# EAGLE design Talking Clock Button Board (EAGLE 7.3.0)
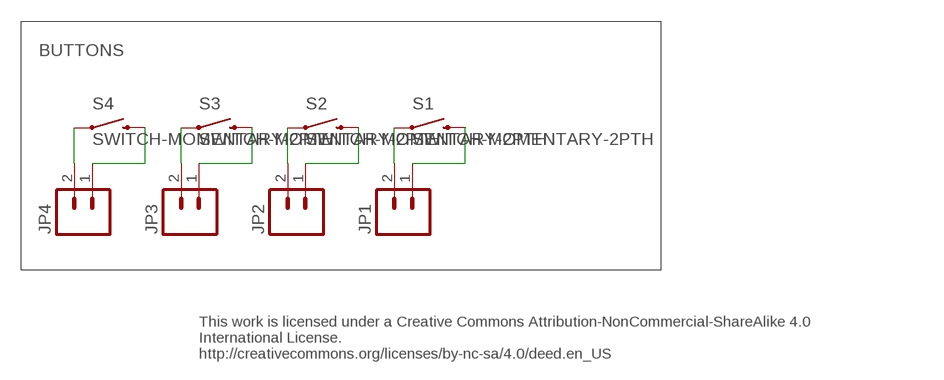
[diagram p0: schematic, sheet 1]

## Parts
JP1  M02PTH  [1X02]
JP2  M02PTH  [1X02]
JP3  M02PTH  [1X02]
JP4  M02PTH  [1X02]
S1  SWITCH-MOMENTARY-2PTH  [TACTILE-PTH]
S2  SWITCH-MOMENTARY-2PTH  [TACTILE-PTH]
S3  SWITCH-MOMENTARY-2PTH  [TACTILE-PTH]
S4  SWITCH-MOMENTARY-2PTH  [TACTILE-PTH]

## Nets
N$1: JP4.2 S4.1
N$2: JP4.1 S4.3
N$3: JP3.2 S3.1
N$4: JP3.1 S3.3
N$5: JP2.2 S2.1
N$6: JP2.1 S2.3
N$7: JP1.2 S1.1
N$8: JP1.1 S1.3

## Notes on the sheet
- BUTTONS
- This work is licensed under a Creative Commons Attribution-NonCommercial-ShareAlike 4.0
  International License.
  http://creativecommons.org/licenses/by-nc-sa/4.0/deed.en_US

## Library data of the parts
JP1-JP4 = SparkFun-Connectors:M02: Standard 2-pin 0.1" header. Use with
S1-S4 = SparkFun-Electromechanical:SWITCH-MOMENTARY-2: Various NO switches- pushbuttons, reed, etc; PROD_ID: SWCH-08441

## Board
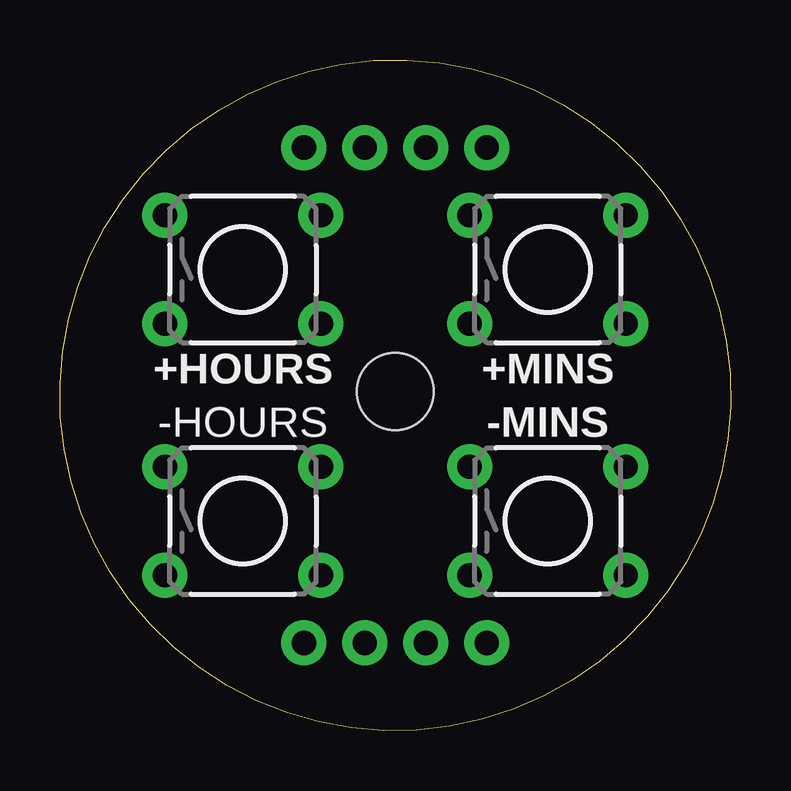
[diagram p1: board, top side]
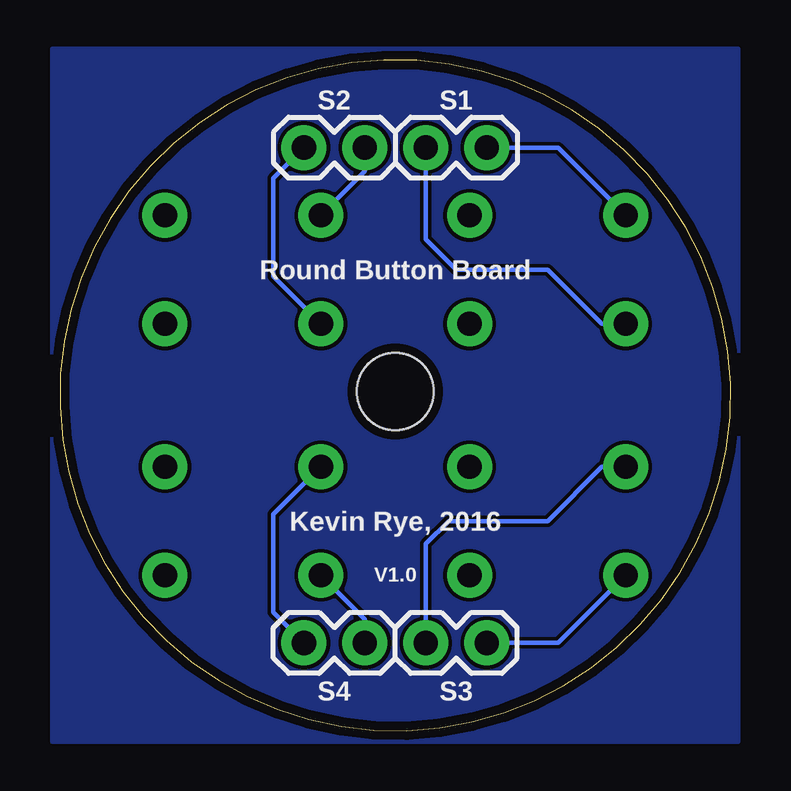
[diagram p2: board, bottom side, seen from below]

Size 27.94 x 27.94 mm. Coordinates in mm from the lower left corner, seen from the top.
Outline: 0,14.45 arc-180 27.94,13.49 arc-180 0,14.45
Copper layers (1*16): Top 0.0356mm / dielectric 1.5011mm / Bottom 0.0356mm
Design rules "oshpark-2layer": minimum track width 6mil, minimum drill 13mil, track to track 6mil, track to pad 6mil, pad to pad 6mil, via to via 6mil, smd to smd 6mil, copper to edge 15mil, drill to drill 6mil, minimum pad ring 7mil, minimum via ring 7mil, stop-mask expansion 2.5mil, vias tented up to drill 0mil, thermal gap 10mil
Holes 3.2 mm at 13.97,14.13

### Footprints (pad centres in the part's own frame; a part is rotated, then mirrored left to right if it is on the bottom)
1X02 = drill 1.016 pad 1.88: 1 0,0; 2 2.54,0
TACTILE-PTH = drill 1.016 pad 1.88: 1 -3.251,2.261; 2 3.251,2.261; 3 -3.251,-2.261; 4 3.251,-2.261

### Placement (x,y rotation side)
JP1  12.7,24.29 0 bottom
JP2  17.78,24.29 0 bottom
JP3  10.16,3.65 180 bottom
JP4  15.24,3.65 180 bottom
S1  7.62,19.21 0 top
S2  20.32,19.21 0 top
S3  7.62,8.73 0 top
S4  20.32,8.73 0 top

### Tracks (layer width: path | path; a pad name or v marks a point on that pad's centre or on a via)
GND
  pour Bottom: -0.32,28.42 28.26,28.42 28.26,-0.48 -0.32,-0.48
N$1
  Bottom 0.178: JP4.2 19.05,4.92 19.05,9.01 S4.1
N$2
  Bottom 0.178: JP4.1 15.24,4.64 S4.3
N$3
  Bottom 0.178: S3.1 5.36,10.99 7.62,8.73 11.75,8.73 12.7,7.78 JP3.2
N$4
  Bottom 0.178: JP3.1 7.19,3.65 S3.3
N$5
  Bottom 0.178: JP2.2 15.24,23.3 S2.1
N$6
  Bottom 0.178: JP2.1 19.05,23.02 19.05,18.93 S2.3
N$7
  Bottom 0.178: JP1.2 7.19,24.29 S1.1
N$8
  Bottom 0.178: S1.3 5.36,16.95 7.62,19.21 11.43,19.21 12.7,20.48 JP1.1

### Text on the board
Unrouted: This work is licensed under a Creative Commons Attribution-NonCommercial-ShareAlike 4.0 International License. / http://creativecommons.org/licenses/by-nc-sa/4.0/deed.en_US
tPlace: +HOURS | +MINS | -HOURS | -MINS
bPlace: S1 | S2 | Round Button Board | Kevin Rye, 2016 | V1.0 | S3 | S4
